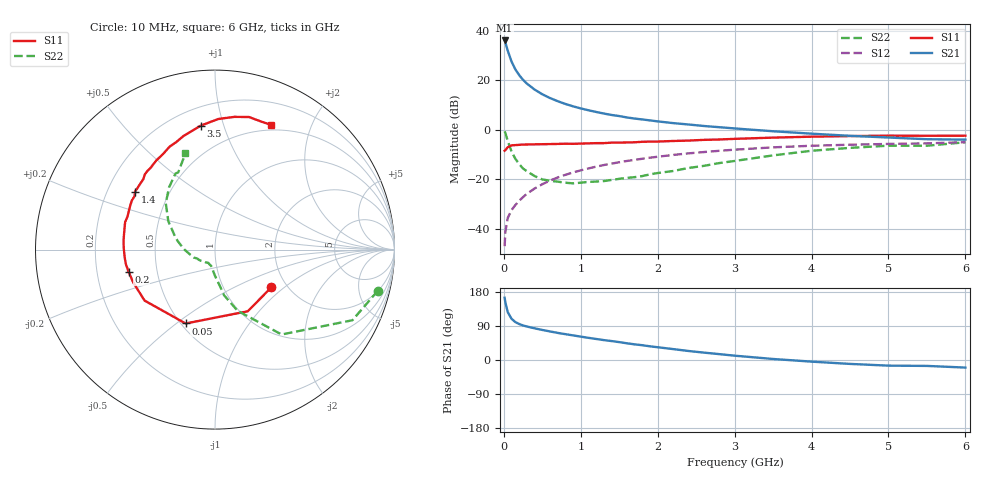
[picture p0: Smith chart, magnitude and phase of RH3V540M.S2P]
! SIEMENS Small Signal Semiconductors
! BFR106
! Si NPN RF Bipolar Junction Transistor in SOT23
! VCE = 3.5 V  IC = 40 mA
! Common Emitter S-Parameters:  August  1996
# GHz  S  MA  R  50
!  f  S11  S21  S12  S22
! GHz  MAG  ANG  MAG  ANG  MAG  ANG  MAG  ANG
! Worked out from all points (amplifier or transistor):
!   36 points, 10 MHz to 6 GHz, reference 50 ohm
!   highest |S21| = 36.2 dB at 10 MHz (marker M1)
!   |S21| within 3 dB of that: start of sweep to 40.13 MHz
!   unconditionally stable (mu >= 1): 268.7 MHz to 2.361 GHz
!   at 250 MHz: K = 0.99, MSG = 23.7 dB, |S12| = -27.2 dB
!   at 1.4 GHz: K = 1.05, MAG = 8.4 dB, |S12| = -13.7 dB
!   at 6 GHz: K = 0.99, MSG = 0.5 dB, |S12| = -5.0 dB
!   S11 on the Smith chart (normalised r, x): 10 MHz: 1.67, -0.82; 50 MHz: 0.53, -0.54; 200 MHz: 0.34, -0.11; 1.4 GHz: 0.32, +0.29; 3.5 GHz: 0.31, +0.84; 6 GHz: 0.44, +1.45
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0.01  0.378 -33.7  64.7 164.3  0.0044 80.6  0.9356 -14.2
0.02  0.3892 -62.0  58.98 151.8  0.0086 72.0  0.8608 -27.2
0.05  0.443 -111.7  40.46 126.6  0.0163 59.9  0.6011 -51.9
0.1  0.4844 -144.1  24.15 108.7  0.0237 59.4  0.3626 -69.8
0.15  0.4913 -158.3  16.74 100.0  0.03 61.5  0.259 -78.8
0.2  0.497 -165.6  12.82 94.9  0.0366 65.5  0.2027 -82.5
0.25  0.5033 -170.9  10.3 91.1  0.0435 66.9  0.1645 -87.0
0.3  0.5049 -175.1  8.631 88.3  0.0507 68.8  0.1449 -90.2
0.4  0.5087 178.9  6.544 83.6  0.0648 69.9  0.1157 -95.9
0.5  0.512 174.1  5.254 79.3  0.0791 70.6  0.0991 -99.9
0.6  0.5146 169.8  4.409 75.4  0.0939 70.1  0.0929 -103.5
0.7  0.5186 166.2  3.807 71.5  0.1084 69.6  0.0892 -108.7
0.9  0.5211 159.2  2.994 64.9  0.1371 67.5  0.0824 -117.2
1.1  0.5319 152.7  2.493 58.5  0.1654 65.2  0.0882 -126.4
1.4  0.5504 144.0  2.003 50.0  0.2069 61.0  0.0966 -138.8
1.7  0.5597 135.5  1.693 41.3  0.2467 56.7  0.1101 -152.5
2.2  0.5947 123.4  1.37 28.8  0.31 49.0  0.1466 -171.4
2.8  0.6376 109.6  1.132 15.5  0.3762 39.6  0.2122 167.3
3.5  0.6956 96.5  0.936 2.7  0.4418 29.0  0.3039 148.8
4.5  0.7474 81.7  0.757 -10.3  0.4995 14.3  0.4312 126.4
5.5  0.7582 69.9  0.646 -15.6  0.5322 4.8  0.4761 115.5
6  0.7618 65.9  0.633 -20.0  0.5634 -2.3  0.5608 107.1
